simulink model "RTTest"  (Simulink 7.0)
settings: Solver=FixedStepDiscrete  StartTime=0.0  StopTime=inf  RelTol=1e-3
PreLoadFcn:
  | samplePeriod = 1/2048;
  | nAct  = 8;
  | nAcc  = 11;
  | nTbl  = 6;
  | nAdcU = 6;
  | 
  | scramInitialize;
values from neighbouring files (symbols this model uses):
  node = scgtnodestruct(node)    [scramInitialize.m]
libraries: cwcec_scgtLib x3, xpclib x2

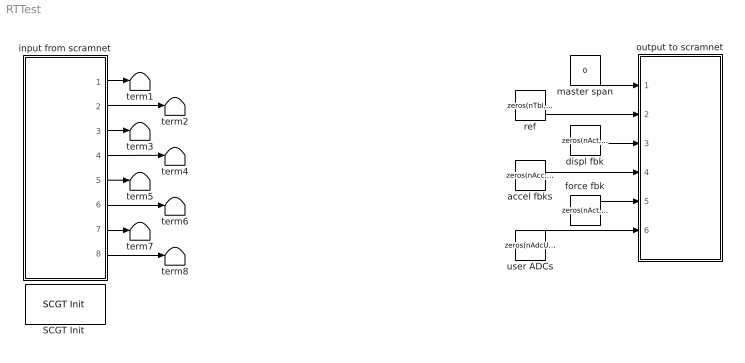
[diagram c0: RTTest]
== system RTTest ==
  "SCGT Init " : cwcec_scgtLib/SCGT Init   node=node  pci=-1
  accel fbks : Constant  Value=zeros(nAcc, 1)  OutDataType=sfix(16)  OutScaling=2^0
  displ fbk : Constant  Value=zeros(nAct, 1)  OutDataType=sfix(16)  OutScaling=2^0
  force fbk : Constant  Value=zeros(nAct, 1)  OutDataType=sfix(16)  OutScaling=2^0
  input from scramnet : Subsystem
  master span : Constant  Value=0  OutDataType=sfix(16)  OutScaling=2^0
  output to scramnet : Subsystem
  ref : Constant  Value=zeros(nTbl, 1)  OutDataType=sfix(16)  OutScaling=2^0
  term{1..8} (8 alike) : Terminator
  user ADCs : Constant  Value=zeros(nAdcU, 1)  OutDataType=sfix(16)  OutScaling=2^0
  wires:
  user ADCs/1 -> output to scramnet/6(user adcs)
  master span/1 -> output to scramnet/1(master span)
  ref/1 -> output to scramnet/2(ref)
  input from scramnet/1(master span) -> term1/1
  input from scramnet/3(displ fbk) -> term3/1
  input from scramnet/4(veloc fbk) -> term4/1
  input from scramnet/6(force fbk) -> term6/1
  input from scramnet/8(user adcs) -> term8/1
  input from scramnet/2(ref) -> term2/1
  input from scramnet/5(accel fbk) -> term5/1
  displ fbk/1 -> output to scramnet/3(displ fbk)
  accel fbks/1 -> output to scramnet/4(accel fbks)
  force fbk/1 -> output to scramnet/5(force fbk)
  input from scramnet/7(valve cmd) -> term7/1

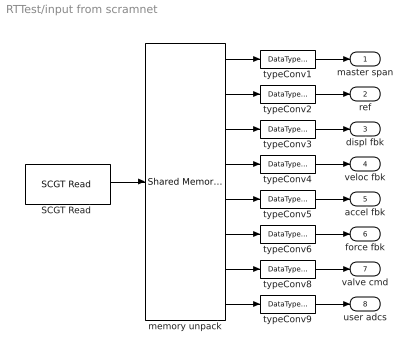
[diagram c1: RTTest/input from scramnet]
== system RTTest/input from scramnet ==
  "SCGT Read " : cwcec_scgtLib/SCGT Read   partition=node.Partitions(7:14)  ts=samplePeriod  pci=-1
  memory unpack : xpclib/Shared Memory/Shared Memory Unpack   partition=node.Partitions(7:14)
  typeConv{1..6,8..9} (8 alike) : DataTypeConversion  OutDataTypeMode=double  OutDataType=sfix(16)  OutScaling=2^0
  master span : Outport  OutDataType=sfix(16)  OutScaling=2^0
  ref : Outport  Port=2  OutDataType=sfix(16)  OutScaling=2^0
  displ fbk : Outport  Port=3  OutDataType=sfix(16)  OutScaling=2^0
  veloc fbk : Outport  Port=4  OutDataType=sfix(16)  OutScaling=2^0
  accel fbk : Outport  Port=5  OutDataType=sfix(16)  OutScaling=2^0
  force fbk : Outport  Port=6  OutDataType=sfix(16)  OutScaling=2^0
  valve cmd : Outport  Port=7  OutDataType=sfix(16)  OutScaling=2^0
  user adcs : Outport  Port=8  OutDataType=sfix(16)  OutScaling=2^0
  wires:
  memory unpack/6 -> typeConv6/1
  memory unpack/5 -> typeConv5/1
  memory unpack/4 -> typeConv4/1
  memory unpack/3 -> typeConv3/1
  memory unpack/7 -> typeConv8/1
  memory unpack/2 -> typeConv2/1
  memory unpack/8 -> typeConv9/1
  memory unpack/1 -> typeConv1/1
  typeConv9/1 -> user adcs/1
  typeConv8/1 -> valve cmd/1
  typeConv6/1 -> force fbk/1
  typeConv5/1 -> accel fbk/1
  typeConv4/1 -> veloc fbk/1
  typeConv3/1 -> displ fbk/1
  typeConv2/1 -> ref/1
  typeConv1/1 -> master span/1
  "SCGT Read "/1 -> memory unpack/1

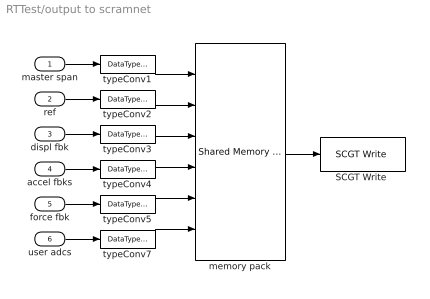
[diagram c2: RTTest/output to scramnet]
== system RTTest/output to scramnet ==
  master span : Inport  OutDataType=sfix(16)  OutScaling=2^0
  ref : Inport  Port=2  OutDataType=sfix(16)  OutScaling=2^0
  displ fbk : Inport  Port=3  OutDataType=sfix(16)  OutScaling=2^0
  accel fbks : Inport  Port=4  OutDataType=sfix(16)  OutScaling=2^0
  force fbk : Inport  Port=5  OutDataType=sfix(16)  OutScaling=2^0
  user adcs : Inport  Port=6  OutDataType=sfix(16)  OutScaling=2^0
  "SCGT Write " : cwcec_scgtLib/SCGT Write   partition=node.Partitions(1:6)  ts=samplePeriod  pci=-1
  memory pack : xpclib/Shared Memory/Shared Memory Pack   partition=node.Partitions(1:6)
  typeConv{1..5,7} (6 alike) : DataTypeConversion  OutDataTypeMode=single  OutDataType=sfix(16)  OutScaling=2^0
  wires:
  typeConv7/1 -> memory pack/6
  typeConv5/1 -> memory pack/5
  user adcs/1 -> typeConv7/1
  force fbk/1 -> typeConv5/1
  typeConv4/1 -> memory pack/4
  typeConv3/1 -> memory pack/3
  typeConv2/1 -> memory pack/2
  typeConv1/1 -> memory pack/1
  memory pack/1 -> "SCGT Write "/1
  accel fbks/1 -> typeConv4/1
  displ fbk/1 -> typeConv3/1
  ref/1 -> typeConv2/1
  master span/1 -> typeConv1/1
